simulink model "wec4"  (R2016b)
settings: Solver=ode4  StartTime=0  StopTime=1000  FixedStep=0.005  MaxStep=0.005  RelTol=1e-3  EnableMultiTasking=on
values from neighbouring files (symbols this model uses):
  arAdaptiveLawData = 1/2*zModelSimple.zModelPto.arFreq.*     zModelSimple.zModelPto.arMagnitude./     cos(zModelSimple.zModelPto.arPhase*pi/180+pi/2)    [IMPACT_Control.m]
  arAdaptiveLawDataX = 1/2*zModelSimpleX.zModelPto.arFreq.*         zModelSimpleX.zModelPto.arMagnitude./         cos(zModelSimpleX.zModelPto.arPhase*pi/180+pi/2)    [IMPACT_Control.m]
  arControllerRampGain = [0,0,1,1]    [IMPACT_Control.m]
  arControllerRampTime = [0 rStartRampTime rStartRampTime+rRampTimeLength 8000]    [IMPACT_Control.m]
  arEkfInitialisation = zeros(1,11)    [IMPACT_Control.m]
  arEkfInitialisationX = zeros(1,11)    [IMPACT_Control.m]
  arFrequency = zModelSimple.zModelPto.arFreq    [IMPACT_Control.m]
  arFrequencyRange = zModelSimple.zModelPto.arFreq    [IMPACT_Control.m]
  arFrequencyX = zModelSimpleX.zModelPto.arFreq    [IMPACT_Control.m]
  arImpedance = 1./zModelSimple.zModelPto.arMagnitude./zModelSimple.zModelPto.arFreq    [IMPACT_Control.m]
  arImpedanceX = 1./zModelSimpleX.zModelPto.arMagnitude./zModelSimpleX.zModelPto.arFreq    [IMPACT_Control.m]
  CentralPTOPreload = -1.6113e+07    (= -16113000)    [wecSimInputFile.m]
  F1 = [4.243 2.375 -12.243]    [wecSimInputFile.m]
  F2 = [4.243 -2.375 -12.243]    [wecSimInputFile.m]
  F3 = [-4.243 -2.375 -12.243]    [wecSimInputFile.m]
  F4 = [-4.243 2.375 -12.243]    [wecSimInputFile.m]
  FC = [0 0 -14]    [wecSimInputFile.m]
  iAdaptiveDamping = 0    [wec4IMPACT_Project.m]    (also in IMPACT_Control.m = handles.iAdaptiveDamping; wec1_IMPACT_Project.m; wec2_IMPACT_Project.m; wec3_IMPACT_Project.m)
  iControlType = 2    [wec4IMPACT_Project.m]    (also in IMPACT_Control.m = handles.iControlType; wec1_IMPACT_Project.m = 1; wec2_IMPACT_Project.m = 1; wec3_IMPACT_Project.m = 1)
  iPtoPositionConstraint = 1    [wec4IMPACT_Project.m]    (also in IMPACT_Control.m = handles.iPtoPositionConstraint; wec1_IMPACT_Project.m = 0; wec2_IMPACT_Project.m; wec3_IMPACT_Project.m)
  iSensorNoise = 0    [IMPACT_Control.m]
  m = m+1    (= 2)    [checkParamFile.m]
  PTOrotation = atan((T1(2)-F1(2))/(T1(1)-F1(1)))    [wecSimInputFile.m]
  rCogFloater = -8    [wec4_IMPACT_Model.m]    (also in paramInitial.m = get( handles.edit_rCogFloater, 'String' ); wec1_IMPACT_Model.m = -18; wec2_IMPACT_Model.m = -8.5; wec3_IMPACT_Model.m = -0.7)
  rCogSpar = -36.6    [wec4_IMPACT_Model.m]    (also in paramInitial.m = get( handles.edit_rCogSpar, 'String' ); wec3_IMPACT_Model.m = -21.3; wec3_IMPACT_Model2.m = -21.3)
  rDisplacementLimit = 10.000000    (= 10)    [wec4IMPACT_Project.m]    (also in IMPACT_Control.m = getValue(handles.edit_displacementLimit); wec1_IMPACT_Project.m; wec2_IMPACT_Project.m; wec3_IMPACT_Project.m = 3)
  rDisplacementLimitX = 10.000000    (= 10)    [wec4IMPACT_Project.m]    (also in IMPACT_Control.m = getValue(handles.edit_displacementLimitX); wec1_IMPACT_Project.m = 0; wec2_IMPACT_Project.m; wec3_IMPACT_Project.m = 0)
  rGainForAntiWIndUp = tfControllerDiscrete.rGain    [IMPACT_Control.m]
  rGainForAntiWIndUpX = tfControllerXDiscrete.rGain    [IMPACT_Control.m]
  rMaxForcePto = 300000000.000000    (= 300000000)    [wec4IMPACT_Project.m]    (also in IMPACT_Control.m = getValue(handles.edit_maxForcePto); wec1_IMPACT_Project.m = 1e+15; wec2_IMPACT_Project.m = 1e+15; wec3_IMPACT_Project.m = 1000000000)
  rMinForcePto = -300000000.000000    (= -300000000)    [wec4IMPACT_Project.m]    (also in IMPACT_Control.m = getValue(handles.edit_minForcePto); wec1_IMPACT_Project.m = -1e+15; wec2_IMPACT_Project.m = -1e+15; wec3_IMPACT_Project.m = -1000000000)
  rMooringX = 20000    [wec4_IMPACT_Model.m]    (also in paramInitial.m = get( handles.edit_rMooringX, 'String' ); wec3_IMPACT_Model.m = 10000; wec3_IMPACT_Model2.m = 10000)
  rMooringZ = 10000    [wec4_IMPACT_Model.m]    (also in paramInitial.m = get( handles.edit_rMooringZ, 'String' ); wec3_IMPACT_Model.m = 0; wec3_IMPACT_Model2.m = 0)
  rOutputSampleTime = 0.010000    (= 0.01)    [wec4IMPACT_Project.m]    (also in IMPACT_Control.m = getValue(handles.edit_outputSampleTime); wec1_IMPACT_Project.m; wec2_IMPACT_Project.m; wec3_IMPACT_Project.m)
  rPassiveDampingGain = -604830.000000    (= -604830)    [wec4IMPACT_Project.m]    (also in IMPACT_Control.m = getValue(handles.edit_gainPLD); wec1_IMPACT_Project.m = -214018.1537; wec2_IMPACT_Project.m = -1948070; wec3_IMPACT_Project.m = -519390)
  rPassiveDampingGainX = -278660.000000    (= -278660)    [wec4IMPACT_Project.m]    (also in IMPACT_Control.m = getValue(handles.edit_gainPLDX); wec1_IMPACT_Project.m = 0; wec2_IMPACT_Project.m = 0; wec3_IMPACT_Project.m = 0)
  rTetherPretension = 1.6113e+07    (= 16113000)    [wec4_IMPACT_Model.m]    (also in paramInitial.m = get( handles.edit_rTetherPretension, 'String' ); wec3_IMPACT_Model.m = 0; wec3_IMPACT_Model2.m = 0)
  rTetherSpring = 500000    [wec4_IMPACT_Model.m]    (also in paramInitial.m = get( handles.edit_rTetherSpring, 'String' ); wec3_IMPACT_Model.m = 0; wec3_IMPACT_Model2.m = 0)
  rUpperFrequencyLimit = EKFFloater.upperFreq    [IMPACT_Control.m]
  rXf = 4.243    [wec4AdditionalParams.m]
  rXs = 16.075    [wec4AdditionalParams.m]
  rYf = 2.375    [wec4AdditionalParams.m]
  rYs = 16.075    [wec4AdditionalParams.m]
  rZf = 4.243    [wec4AdditionalParams.m]
  rZs = 2.4350    (= 2.435)    [wec4AdditionalParams.m]
  rZTetherF = 6    [wec4AdditionalParams.m]
  rZTetherS = 2.4350    (= 2.435)    [wec4AdditionalParams.m]
  s = tf('s')    [wec4_IMPACT_Model.m]    (also in IMPACT_Control.m; wec1_IMPACT_Model.m; wec2_IMPACT_Model.m; wec3_IMPACT_Model.m)
  SidePTO1Preload = PreloadPTOCorner    (= 0)    [wecSimInputFile.m]
  SidePTO2Preload = PreloadPTOCorner    (= 0)    [wecSimInputFile.m]
  SidePTO3Preload = PreloadPTOCorner    (= 0)    [wecSimInputFile.m]
  SidePTO4Preload = PreloadPTOCorner    (= 0)    [wecSimInputFile.m]
  simu = simulationClass()    [wecSimInputFile.m]
  T1 = [16.075 16.075 -34.165]    [wecSimInputFile.m]
  T2 = [16.075 -16.075 -34.165]    [wecSimInputFile.m]
  T3 = [-16.075 -16.075 -34.165]    [wecSimInputFile.m]
  T4 = [-16.075 16.075 -34.165]    [wecSimInputFile.m]
  TC = [0 0 -34.165]    [wecSimInputFile.m]
  waves = waveClass('irregular')    [wecSimInputFile.m]
  Z = magPhaseToComplex(zModelTf)    [IMPACT_Control.m]
undefined symbols (not defined in the file or in its folder): arControllerDiscreteDen, arControllerDiscreteNum, arControllerDiscreteXDen, arControllerDiscreteXNum, arExcForceFloaterDen, arExcForceFloaterNum, arExcForceFloaterXDen, arExcForceFloaterXNum, arExcForceSparDen, arExcForceSparNum, arExcForceSparXDen, arExcForceSparXNum, arFexcFloaterDen, arFexcFloaterNum, arFexcFloaterXDen, arFexcFloaterXNum, arFexcSparDen, arFexcSparNum, arFexcSparXDen, arFexcSparXNum, Body, body, constraint, CTTime, deg, Elements, geometry, IRKB, kg, lenJ, mooring, N, pto, rAccelerationGainFloater, rAccelerationGainFloaterX, rAccelerationGainSpar, rAccelerationGainSparX, rad, rBuoyancyGainFloater, rBuoyancyGainFloaterX, rBuoyancyGainSpar, rBuoyancyGainSparX, rDampingGainFloater, rDampingGainFloaterX, rDampingGainSpar, rDampingGainSparX, Rigid, rMaxFocePto, wec4_float, wec4_reactor, WECSim_Lib, X, Y
libraries: nesl_utility x380, sm_lib x170, vrlib x91, simulink x12, WECSim_Lib x4
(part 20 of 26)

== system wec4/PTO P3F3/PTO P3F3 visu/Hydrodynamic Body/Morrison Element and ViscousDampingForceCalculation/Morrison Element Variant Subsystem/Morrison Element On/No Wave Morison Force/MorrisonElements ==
  r : Inport  Partition=on  PartitionDimension=1  PartitionWidth=1
  Vel : Inport  Port=2
  Accel : Inport  Port=3
  Disp : Inport  Port=4
  Area : Inport  Port=5  Partition=on  PartitionDimension=1  PartitionWidth=1
  Cd : Inport  Port=6  Partition=on  PartitionDimension=1  PartitionWidth=1
  Vol : Inport  Port=7  Partition=on  PartitionDimension=1  PartitionWidth=1
  Ca : Inport  Port=8  Partition=on  PartitionDimension=1  PartitionWidth=1
  Time : Inport  Port=9
  3x3 : Concatenate  NumInputs=3  Mode=Multidimensional array
  A x 3x3 : Product  Multiplication=Matrix(*)
  Accel-sl : Selector  InputPortWidth=6  IndexOptions=Index vector (dialog)  Indices=[1 2 3]  OutputSizes=1
  Accel-sr : Selector  InputPortWidth=6  IndexOptions=Index vector (dialog)  Indices=[4 5 6]  OutputSizes=1
  AccelDiff-u : Sum  Inputs=+-
  AccelDiff-v : Sum  Inputs=+-
  AccelDiff-w : Sum  Inputs=+-
  Add Accel : Sum  Inputs=+++
  Add Vel : Sum
  Ax : Selector  InputPortWidth=3  IndexOptions=Index vector (dialog)  Indices=[1]  OutputSizes=1
  Ay : Selector  InputPortWidth=3  IndexOptions=Index vector (dialog)  Indices=[2]  OutputSizes=1
  Az : Selector  InputPortWidth=3  IndexOptions=Index vector (dialog)  Indices=[3]  OutputSizes=1
  Cax : Selector  InputPortWidth=3  IndexOptions=Index vector (dialog)  Indices=[1]  OutputSizes=1
  Cay : Selector  InputPortWidth=3  IndexOptions=Index vector (dialog)  Indices=[2]  OutputSizes=1
  Caz : Selector  InputPortWidth=3  IndexOptions=Index vector (dialog)  Indices=[3]  OutputSizes=1
  Cdx : Selector  InputPortWidth=3  IndexOptions=Index vector (dialog)  Indices=[1]  OutputSizes=1
  Cdy : Selector  InputPortWidth=3  IndexOptions=Index vector (dialog)  Indices=[2]  OutputSizes=1
  Cdz : Selector  InputPortWidth=3  IndexOptions=Index vector (dialog)  Indices=[3]  OutputSizes=1
  Constant : Constant  Value=0
  Density : Constant  Value=simu.rho
  Disp-sl : Selector  InputPortWidth=6  IndexOptions=Index vector (dialog)  Indices=[1 2 3]  OutputSizes=1
  Disp-sr : Selector  InputPortWidth=6  IndexOptions=Index vector (dialog)  Indices=[4 5 6]  OutputSizes=1
  For Each : ForEach  DisableCoverage=on  IndexMode=One-based
  ForceCom : Concatenate  NumInputs=3  ConcatenateDimension=2
  Fout : Concatenate  NumInputs=6  Mode=Multidimensional array  ConcatenateDimension=2
  Fx-A : Product  Inputs=4
  Fx-AFK : Product  Inputs=3
  Fx-Sum : Sum  Inputs=+++
  Fx-V : Product  Inputs=5
  Fx-V1 : Product  Inputs=5
  Fy-A : Product  Inputs=4
  Fy-AFK : Product  Inputs=3
  Fy-Sum : Sum  Inputs=+++
  Fz-A : Product  Inputs=4
  Fz-AFK : Product  Inputs=3
  Fz-Sum : Sum  Inputs=+++
  Fz-w : Product  Inputs=5
  Mx : Selector  InputPortWidth=3  IndexOptions=Index vector (dialog)  Indices=[1]  OutputSizes=1
  My : Selector  InputPortWidth=3  IndexOptions=Index vector (dialog)  Indices=[2]  OutputSizes=1
  Mz : Selector  InputPortWidth=3  IndexOptions=Index vector (dialog)  Indices=[3]  OutputSizes=1
  OrbitalVelocity : Subsystem
  Rotation1 : Subsystem
  Rotation2 : Subsystem
  Rotation3 : Subsystem
  ShiftCg : Sum
  SwitchFx : Switch  Criteria=u2 > Threshold
  SwitchFy : Switch  Criteria=u2 > Threshold
  SwitchFz : Switch  Criteria=u2 > Threshold
  Ux : Selector  InputPortWidth=3  IndexOptions=Index vector (dialog)  Indices=[1]  OutputSizes=1
  Uy : Selector  InputPortWidth=3  IndexOptions=Index vector (dialog)  Indices=[2]  OutputSizes=1
  Uz : Selector  InputPortWidth=3  IndexOptions=Index vector (dialog)  Indices=[3]  OutputSizes=1
  V-u : Abs
  V-v : Abs
  V-w : Abs
  V^2-u : Product
  V^2-v : Product
  V^2-w : Product
  Vel-sl : Selector  InputPortWidth=6  IndexOptions=Index vector (dialog)  Indices=[1 2 3]  OutputSizes=1
  "Vel-sr " : Selector  InputPortWidth=6  IndexOptions=Index vector (dialog)  Indices=[4 5 6]  OutputSizes=1
  VelDiff-u : Sum  Inputs=+-
  VelDiff-v : Sum  Inputs=+-
  VelDiff-w : Sum  Inputs=+-
  Zshift : Selector  InputPortWidth=3  IndexOptions=Index vector (dialog)  Indices=[3]  OutputSizes=1
  abs-Area : Abs
  abs-Ca : Abs
  abs-Cd : Abs
  "dot{U}x" : Selector  InputPortWidth=3  IndexOptions=Index vector (dialog)  Indices=[1]  OutputSizes=1
  "dot{U}y" : Selector  InputPortWidth=3  IndexOptions=Index vector (dialog)  Indices=[2]  OutputSizes=1
  "dot{U}z" : Selector  InputPortWidth=3  IndexOptions=Index vector (dialog)  Indices=[3]  OutputSizes=1
  "dot{w} x r2" : vrlib/Utilities/Cross Product
  half : Constant  Value=1/2
  r x 3x1 : Product  Multiplication=Matrix(*)
  r x 3x2 : Product  Multiplication=Matrix(*)
  r x 3x3 : Product  Multiplication=Matrix(*)
  "r_{cg} x F" : vrlib/Utilities/Cross Product
  rot1 : Selector  InputPortWidth=3  IndexOptions=Index vector (dialog)  Indices=[1]  OutputSizes=1
  rot2 : Selector  InputPortWidth=3  IndexOptions=Index vector (dialog)  Indices=[2]  OutputSizes=1
  rot3 : Selector  InputPortWidth=3  IndexOptions=Index vector (dialog)  Indices=[3]  OutputSizes=1
  w x r : vrlib/Utilities/Cross Product
  w x w x r : vrlib/Utilities/Cross Product
  Force : Outport  PortDimensions=[1 6]  ConcatenationDimension=1
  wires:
  Time/1 -> OrbitalVelocity/2(Time)
  abs-Cd/1 -> r x 3x1/1
  abs-Ca/1 -> Caz/1, Cay/1, Cax/1
  V-w/1 -> V^2-w/1
  Constant/1 -> SwitchFx/1, SwitchFz/1, SwitchFy/1
  Fx-V1/1 -> Fy-Sum/1
  Fy-A/1 -> Fy-Sum/2
  Cay/1 -> Fy-A/4
  AccelDiff-v/1 -> Fy-A/1
  Fy-AFK/1 -> Fy-Sum/3
  Fy-Sum/1 -> SwitchFy/3
  SwitchFy/1 -> ForceCom/2, Fout/2
  Cdy/1 -> Fx-V1/4
  Ay/1 -> Fx-V1/5
  OrbitalVelocity/5(v-V) -> VelDiff-v/1
  VelDiff-v/1 -> V^2-v/2, V-v/1
  V-v/1 -> V^2-v/1
  V^2-v/1 -> Fx-V1/1
  OrbitalVelocity/6(v-A) -> Fy-AFK/1, AccelDiff-v/1
  r x 3x2/1 -> abs-Ca/1
  Ca/1 -> r x 3x2/1
  r x 3x1/1 -> Cdx/1, Cdz/1, Cdy/1
  Cd/1 -> abs-Cd/1
  Cax/1 -> Fx-A/4
  Caz/1 -> Fz-A/4
  Fout/1 -> Force/1
  ForceCom/1 -> "r_{cg} x F"/2
  abs-Area/1 -> Ax/1, Az/1, Ay/1
  A x 3x3/1 -> abs-Area/1
  Cdz/1 -> Fz-w/4
  Cdx/1 -> Fx-V/4
  Ax/1 -> Fx-V/5
  Area/1 -> A x 3x3/1
  Az/1 -> Fz-w/5
  Fz-Sum/1 -> SwitchFz/3
  Fx-Sum/1 -> SwitchFx/3
  SwitchFx/1 -> ForceCom/1, Fout/1
  SwitchFz/1 -> Fout/3, ForceCom/3
  Zshift/1 -> SwitchFz/2, SwitchFx/2, SwitchFy/2
  VelDiff-u/1 -> V^2-u/2, V-u/1
  V-u/1 -> V^2-u/1
  3x3/1 -> r x 3x1/2, r x 3x2/2, r x 3x3/2, A x 3x3/2
  Mz/1 -> Fout/6
  My/1 -> Fout/5
  Mx/1 -> Fout/4
  "r_{cg} x F"/1 -> Mx/1, My/1, Mz/1
  Fz-AFK/1 -> Fz-Sum/3
  Fz-A/1 -> Fz-Sum/2
  Fz-w/1 -> Fz-Sum/1
  Fx-AFK/1 -> Fx-Sum/3
  Fx-A/1 -> Fx-Sum/2
  Fx-V/1 -> Fx-Sum/1
  OrbitalVelocity/4(w-A) -> AccelDiff-w/1, Fz-AFK/1
  AccelDiff-w/1 -> Fz-A/1
  Vol/1 -> Fx-A/3, Fz-A/2, Fx-AFK/2, Fz-AFK/2, Fy-AFK/2, Fy-A/2
  AccelDiff-u/1 -> Fx-A/1
  V^2-w/1 -> Fz-w/1
  Density/1 -> Fx-V/3, Fx-V1/3, Fz-w/3, Fx-A/2, Fz-A/3, Fx-AFK/3, Fz-AFK/3, Fy-AFK/3, Fy-A/3
  half/1 -> Fx-V/2, Fx-V1/2, Fz-w/2
  V^2-u/1 -> Fx-V/1
  VelDiff-w/1 -> V^2-w/2, V-w/1
  OrbitalVelocity/2(w-V) -> VelDiff-w/1
  OrbitalVelocity/1(u-V) -> VelDiff-u/1
  Uz/1 -> VelDiff-w/2
  Ux/1 -> VelDiff-u/2
  Uy/1 -> VelDiff-v/2
  Add Vel/1 -> Ux/1, Uz/1, Uy/1
  "dot{U}z"/1 -> AccelDiff-w/2
  OrbitalVelocity/3(u-A) -> Fx-AFK/1, AccelDiff-u/1
  "dot{U}x"/1 -> AccelDiff-u/2
  "dot{U}y"/1 -> AccelDiff-v/2
  ShiftCg/1 -> OrbitalVelocity/1(Disp), Zshift/1
  Disp-sl/1 -> ShiftCg/2
  r x 3x3/1 -> ShiftCg/1, "r_{cg} x F"/1
  Rotation3/1(rot[3,1-3]) -> 3x3/3
  Rotation1/1(rot[1,1-3]) -> 3x3/1
  Rotation2/1(rot[2,1-3]) -> 3x3/2
  rot2/1 -> Rotation1/2(rot2), Rotation2/2(rot2), Rotation3/2(rot2)
  rot1/1 -> Rotation1/1(rot1), Rotation2/1(rot1), Rotation3/1(rot1)
  rot3/1 -> Rotation1/3(rot3), Rotation2/3(rot3)
  Disp-sr/1 -> rot1/1, rot2/1, rot3/1
  Disp/1 -> Disp-sr/1, Disp-sl/1
  Vel-sl/1 -> Add Vel/1
  Add Accel/1 -> "dot{U}x"/1, "dot{U}y"/1, "dot{U}z"/1
  Accel-sl/1 -> Add Accel/3
  "dot{w} x r2"/1 -> Add Accel/2
  Accel-sr/1 -> "dot{w} x r2"/1
  Accel/1 -> Accel-sr/1, Accel-sl/1
  r/1 -> w x r/2, "dot{w} x r2"/2, r x 3x3/1
  "Vel-sr "/1 -> w x r/1, w x w x r/1
  w x w x r/1 -> Add Accel/1
  w x r/1 -> w x w x r/2, Add Vel/2
  Vel/1 -> "Vel-sr "/1, Vel-sl/1

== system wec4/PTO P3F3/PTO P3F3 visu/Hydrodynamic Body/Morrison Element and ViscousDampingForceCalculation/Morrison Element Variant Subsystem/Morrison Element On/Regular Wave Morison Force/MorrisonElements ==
  r : Inport  Partition=on  PartitionDimension=1  PartitionWidth=1
  Vel : Inport  Port=2
  Accel : Inport  Port=3
  Disp : Inport  Port=4
  Area : Inport  Port=5  Partition=on  PartitionDimension=1  PartitionWidth=1
  Cd : Inport  Port=6  Partition=on  PartitionDimension=1  PartitionWidth=1
  Vol : Inport  Port=7  Partition=on  PartitionDimension=1  PartitionWidth=1
  Ca : Inport  Port=8  Partition=on  PartitionDimension=1  PartitionWidth=1
  Time : Inport  Port=9
  3x3 : Concatenate  NumInputs=3  Mode=Multidimensional array
  A x 3x3 : Product  Multiplication=Matrix(*)
  Accel-sl : Selector  InputPortWidth=6  IndexOptions=Index vector (dialog)  Indices=[1 2 3]  OutputSizes=1
  Accel-sr : Selector  InputPortWidth=6  IndexOptions=Index vector (dialog)  Indices=[4 5 6]  OutputSizes=1
  AccelDiff-u : Sum  Inputs=+-
  AccelDiff-v : Sum  Inputs=+-
  AccelDiff-w : Sum  Inputs=+-
  Add Accel : Sum  Inputs=+++
  Add Vel : Sum
  Ax : Selector  InputPortWidth=3  IndexOptions=Index vector (dialog)  Indices=[1]  OutputSizes=1
  Ay : Selector  InputPortWidth=3  IndexOptions=Index vector (dialog)  Indices=[2]  OutputSizes=1
  Az : Selector  InputPortWidth=3  IndexOptions=Index vector (dialog)  Indices=[3]  OutputSizes=1
  Cax : Selector  InputPortWidth=3  IndexOptions=Index vector (dialog)  Indices=[1]  OutputSizes=1
  Cay : Selector  InputPortWidth=3  IndexOptions=Index vector (dialog)  Indices=[2]  OutputSizes=1
  Caz : Selector  InputPortWidth=3  IndexOptions=Index vector (dialog)  Indices=[3]  OutputSizes=1
  Cdx : Selector  InputPortWidth=3  IndexOptions=Index vector (dialog)  Indices=[1]  OutputSizes=1
  Cdy : Selector  InputPortWidth=3  IndexOptions=Index vector (dialog)  Indices=[2]  OutputSizes=1
  Cdz : Selector  InputPortWidth=3  IndexOptions=Index vector (dialog)  Indices=[3]  OutputSizes=1
  Constant : Constant  Value=0
  Density : Constant  Value=simu.rho
  Disp-sl : Selector  InputPortWidth=6  IndexOptions=Index vector (dialog)  Indices=[1 2 3]  OutputSizes=1
  Disp-sr : Selector  InputPortWidth=6  IndexOptions=Index vector (dialog)  Indices=[4 5 6]  OutputSizes=1
  For Each : ForEach  DisableCoverage=on  IndexMode=One-based
  ForceCom : Concatenate  NumInputs=3  ConcatenateDimension=2
  Fout : Concatenate  NumInputs=6  Mode=Multidimensional array  ConcatenateDimension=2
  Fx-A : Product  Inputs=4
  Fx-AFK : Product  Inputs=3
  Fx-Sum : Sum  Inputs=+++
  Fx-V : Product  Inputs=5
  Fx-V1 : Product  Inputs=5
  Fy-A : Product  Inputs=4
  Fy-AFK : Product  Inputs=3
  Fy-Sum : Sum  Inputs=+++
  Fz-A : Product  Inputs=4
  Fz-AFK : Product  Inputs=3
  Fz-Sum : Sum  Inputs=+++
  Fz-w : Product  Inputs=5
  Mx : Selector  InputPortWidth=3  IndexOptions=Index vector (dialog)  Indices=[1]  OutputSizes=1
  My : Selector  InputPortWidth=3  IndexOptions=Index vector (dialog)  Indices=[2]  OutputSizes=1
  Mz : Selector  InputPortWidth=3  IndexOptions=Index vector (dialog)  Indices=[3]  OutputSizes=1
  OrbitalVelocity : Subsystem
  Rotation1 : Subsystem
  Rotation2 : Subsystem
  Rotation3 : Subsystem
  ShiftCg : Sum
  SwitchFx : Switch  Criteria=u2 > Threshold
  SwitchFy : Switch  Criteria=u2 > Threshold
  SwitchFz : Switch  Criteria=u2 > Threshold
  Ux : Selector  InputPortWidth=3  IndexOptions=Index vector (dialog)  Indices=[1]  OutputSizes=1
  Uy : Selector  InputPortWidth=3  IndexOptions=Index vector (dialog)  Indices=[2]  OutputSizes=1
  Uz : Selector  InputPortWidth=3  IndexOptions=Index vector (dialog)  Indices=[3]  OutputSizes=1
  V-u : Abs
  V-v : Abs
  V-w : Abs
  V^2-u : Product
  V^2-v : Product
  V^2-w : Product
  Vel-sl : Selector  InputPortWidth=6  IndexOptions=Index vector (dialog)  Indices=[1 2 3]  OutputSizes=1
  "Vel-sr " : Selector  InputPortWidth=6  IndexOptions=Index vector (dialog)  Indices=[4 5 6]  OutputSizes=1
  VelDiff-u : Sum  Inputs=+-
  VelDiff-v : Sum  Inputs=+-
  VelDiff-w : Sum  Inputs=+-
  Zshift : Selector  InputPortWidth=3  IndexOptions=Index vector (dialog)  Indices=[3]  OutputSizes=1
  abs-Area : Abs
  abs-Ca : Abs
  abs-Cd : Abs
  "dot{U}x" : Selector  InputPortWidth=3  IndexOptions=Index vector (dialog)  Indices=[1]  OutputSizes=1
  "dot{U}y" : Selector  InputPortWidth=3  IndexOptions=Index vector (dialog)  Indices=[2]  OutputSizes=1
  "dot{U}z" : Selector  InputPortWidth=3  IndexOptions=Index vector (dialog)  Indices=[3]  OutputSizes=1
  "dot{w} x r2" : vrlib/Utilities/Cross Product
  half : Constant  Value=1/2
  r x 3x1 : Product  Multiplication=Matrix(*)
  r x 3x2 : Product  Multiplication=Matrix(*)
  r x 3x3 : Product  Multiplication=Matrix(*)
  "r_{cg} x F" : vrlib/Utilities/Cross Product
  rot1 : Selector  InputPortWidth=3  IndexOptions=Index vector (dialog)  Indices=[1]  OutputSizes=1
  rot2 : Selector  InputPortWidth=3  IndexOptions=Index vector (dialog)  Indices=[2]  OutputSizes=1
  rot3 : Selector  InputPortWidth=3  IndexOptions=Index vector (dialog)  Indices=[3]  OutputSizes=1
  w x r : vrlib/Utilities/Cross Product
  w x w x r : vrlib/Utilities/Cross Product
  Force : Outport  PortDimensions=[1 6]  ConcatenationDimension=1
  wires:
  Time/1 -> OrbitalVelocity/2(Time)
  abs-Cd/1 -> r x 3x1/1
  abs-Ca/1 -> Caz/1, Cay/1, Cax/1
  V-w/1 -> V^2-w/1
  Constant/1 -> SwitchFx/1, SwitchFz/1, SwitchFy/1
  Fx-V1/1 -> Fy-Sum/1
  Fy-A/1 -> Fy-Sum/2
  Cay/1 -> Fy-A/4
  AccelDiff-v/1 -> Fy-A/1
  Fy-AFK/1 -> Fy-Sum/3
  Fy-Sum/1 -> SwitchFy/3
  SwitchFy/1 -> ForceCom/2, Fout/2
  Cdy/1 -> Fx-V1/4
  Ay/1 -> Fx-V1/5
  OrbitalVelocity/5(v-V) -> VelDiff-v/1
  VelDiff-v/1 -> V^2-v/2, V-v/1
  V-v/1 -> V^2-v/1
  V^2-v/1 -> Fx-V1/1
  OrbitalVelocity/6(v-A) -> Fy-AFK/1, AccelDiff-v/1
  r x 3x2/1 -> abs-Ca/1
  Ca/1 -> r x 3x2/1
  r x 3x1/1 -> Cdx/1, Cdz/1, Cdy/1
  Cd/1 -> abs-Cd/1
  Cax/1 -> Fx-A/4
  Caz/1 -> Fz-A/4
  Fout/1 -> Force/1
  ForceCom/1 -> "r_{cg} x F"/2
  abs-Area/1 -> Ax/1, Az/1, Ay/1
  A x 3x3/1 -> abs-Area/1
  Cdz/1 -> Fz-w/4
  Cdx/1 -> Fx-V/4
  Ax/1 -> Fx-V/5
  Area/1 -> A x 3x3/1
  Az/1 -> Fz-w/5
  Fz-Sum/1 -> SwitchFz/3
  Fx-Sum/1 -> SwitchFx/3
  SwitchFx/1 -> ForceCom/1, Fout/1
  SwitchFz/1 -> Fout/3, ForceCom/3
  Zshift/1 -> SwitchFz/2, SwitchFx/2, SwitchFy/2
  VelDiff-u/1 -> V^2-u/2, V-u/1
  V-u/1 -> V^2-u/1
  3x3/1 -> r x 3x1/2, r x 3x2/2, r x 3x3/2, A x 3x3/2
  Mz/1 -> Fout/6
  My/1 -> Fout/5
  Mx/1 -> Fout/4
  "r_{cg} x F"/1 -> Mx/1, My/1, Mz/1
  Fz-AFK/1 -> Fz-Sum/3
  Fz-A/1 -> Fz-Sum/2
  Fz-w/1 -> Fz-Sum/1
  Fx-AFK/1 -> Fx-Sum/3
  Fx-A/1 -> Fx-Sum/2
  Fx-V/1 -> Fx-Sum/1
  OrbitalVelocity/4(w-A) -> AccelDiff-w/1, Fz-AFK/1
  AccelDiff-w/1 -> Fz-A/1
  Vol/1 -> Fx-A/3, Fz-A/2, Fx-AFK/2, Fz-AFK/2, Fy-AFK/2, Fy-A/2
  AccelDiff-u/1 -> Fx-A/1
  V^2-w/1 -> Fz-w/1
  Density/1 -> Fx-V/3, Fx-V1/3, Fz-w/3, Fx-A/2, Fz-A/3, Fx-AFK/3, Fz-AFK/3, Fy-AFK/3, Fy-A/3
  half/1 -> Fx-V/2, Fx-V1/2, Fz-w/2
  V^2-u/1 -> Fx-V/1
  VelDiff-w/1 -> V^2-w/2, V-w/1
  OrbitalVelocity/2(w-V) -> VelDiff-w/1
  OrbitalVelocity/1(u-V) -> VelDiff-u/1
  Uz/1 -> VelDiff-w/2
  Ux/1 -> VelDiff-u/2
  Uy/1 -> VelDiff-v/2
  Add Vel/1 -> Ux/1, Uz/1, Uy/1
  "dot{U}z"/1 -> AccelDiff-w/2
  OrbitalVelocity/3(u-A) -> Fx-AFK/1, AccelDiff-u/1
  "dot{U}x"/1 -> AccelDiff-u/2
  "dot{U}y"/1 -> AccelDiff-v/2
  ShiftCg/1 -> OrbitalVelocity/1(Disp), Zshift/1
  Disp-sl/1 -> ShiftCg/2
  r x 3x3/1 -> ShiftCg/1, "r_{cg} x F"/1
  Rotation3/1(rot[3,1-3]) -> 3x3/3
  Rotation1/1(rot[1,1-3]) -> 3x3/1
  Rotation2/1(rot[2,1-3]) -> 3x3/2
  rot2/1 -> Rotation1/2(rot2), Rotation2/2(rot2), Rotation3/2(rot2)
  rot1/1 -> Rotation1/1(rot1), Rotation2/1(rot1), Rotation3/1(rot1)
  rot3/1 -> Rotation1/3(rot3), Rotation2/3(rot3)
  Disp-sr/1 -> rot1/1, rot2/1, rot3/1
  Disp/1 -> Disp-sr/1, Disp-sl/1
  Vel-sl/1 -> Add Vel/1
  Add Accel/1 -> "dot{U}x"/1, "dot{U}y"/1, "dot{U}z"/1
  Accel-sl/1 -> Add Accel/3
  "dot{w} x r2"/1 -> Add Accel/2
  Accel-sr/1 -> "dot{w} x r2"/1
  Accel/1 -> Accel-sr/1, Accel-sl/1
  r/1 -> w x r/2, "dot{w} x r2"/2, r x 3x3/1
  "Vel-sr "/1 -> w x r/1, w x w x r/1
  w x w x r/1 -> Add Accel/1
  w x r/1 -> w x w x r/2, Add Vel/2
  Vel/1 -> "Vel-sr "/1, Vel-sl/1

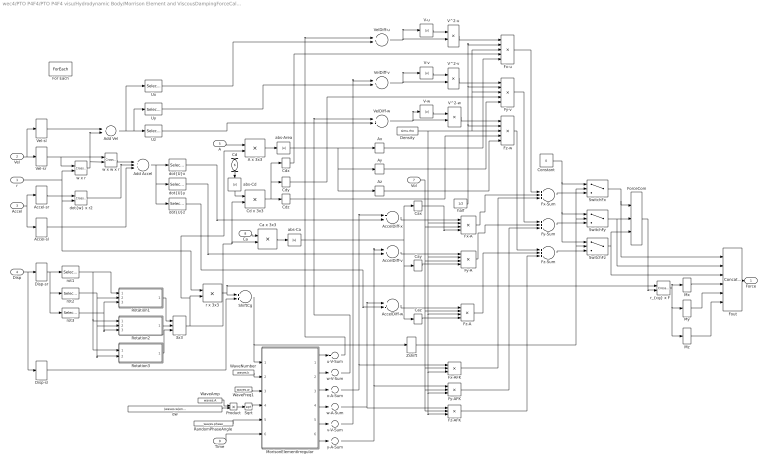
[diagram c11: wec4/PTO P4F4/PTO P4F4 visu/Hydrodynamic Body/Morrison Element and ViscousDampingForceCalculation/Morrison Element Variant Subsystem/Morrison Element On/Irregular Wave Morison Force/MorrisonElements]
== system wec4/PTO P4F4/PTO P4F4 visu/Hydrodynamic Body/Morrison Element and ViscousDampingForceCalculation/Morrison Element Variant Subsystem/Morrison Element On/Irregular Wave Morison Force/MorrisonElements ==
  r : Inport  Partition=on  PartitionDimension=1  PartitionWidth=1
  Vel : Inport  Port=2
  Accel : Inport  Port=3
  Disp : Inport  Port=4
  A : Inport  Port=5  Partition=on  PartitionDimension=1  PartitionWidth=1
  Cd : Inport  Port=6  Partition=on  PartitionDimension=1  PartitionWidth=1
  Vol : Inport  Port=7  Partition=on  PartitionDimension=1  PartitionWidth=1
  Ca : Inport  Port=8  Partition=on  PartitionDimension=1  PartitionWidth=1
  Time : Inport  Port=9
  3x3 : Concatenate  NumInputs=3  Mode=Multidimensional array
  A x 3x3 : Product  Multiplication=Matrix(*)
  Accel-sl : Selector  InputPortWidth=6  IndexOptions=Index vector (dialog)  Indices=[1 2 3]  OutputSizes=1
  Accel-sr : Selector  InputPortWidth=6  IndexOptions=Index vector (dialog)  Indices=[4 5 6]  OutputSizes=1
  AccelDiff-v : Sum  Inputs=+-
  AccelDiff-w : Sum  Inputs=+-
  AccelDiff-x : Sum  Inputs=+-
  Add Accel : Sum  Inputs=+++
  Add Vel : Sum
  Ax : Selector  InputPortWidth=3  IndexOptions=Index vector (dialog)  Indices=[1]  OutputSizes=1
  Ay : Selector  InputPortWidth=3  IndexOptions=Index vector (dialog)  Indices=[2]  OutputSizes=1
  Az : Selector  InputPortWidth=3  IndexOptions=Index vector (dialog)  Indices=[3]  OutputSizes=1
  Ca x 3x3 : Product  Multiplication=Matrix(*)
  Cax : Selector  InputPortWidth=3  IndexOptions=Index vector (dialog)  Indices=[1]  OutputSizes=1
  Cay : Selector  InputPortWidth=3  IndexOptions=Index vector (dialog)  Indices=[2]  OutputSizes=1
  Caz : Selector  InputPortWidth=3  IndexOptions=Index vector (dialog)  Indices=[3]  OutputSizes=1
  Cd x 3x3 : Product  Multiplication=Matrix(*)
  Cdx : Selector  InputPortWidth=3  IndexOptions=Index vector (dialog)  Indices=[1]  OutputSizes=1
  Cdy : Selector  InputPortWidth=3  IndexOptions=Index vector (dialog)  Indices=[2]  OutputSizes=1
  Cdz : Selector  InputPortWidth=3  IndexOptions=Index vector (dialog)  Indices=[3]  OutputSizes=1
  Constant : Constant  Value=0
  Density : Constant  Value=simu.rho
  Disp-sl : Selector  InputPortWidth=6  IndexOptions=Index vector (dialog)  Indices=[1 2 3]  OutputSizes=1
  Disp-sr : Selector  InputPortWidth=6  IndexOptions=Index vector (dialog)  Indices=[4 5 6]  OutputSizes=1
  For Each : ForEach  DisableCoverage=on  IndexMode=One-based
  ForceCom : Concatenate  NumInputs=3  ConcatenateDimension=2
  Fout : Concatenate  NumInputs=6  Mode=Multidimensional array  ConcatenateDimension=2
  Fx-A : Product  Inputs=4
  Fx-AFK : Product  Inputs=3
  Fx-Sum : Sum  Inputs=+++
  Fx-u : Product  Inputs=5
  Fy-A : Product  Inputs=4
  Fy-AFK : Product  Inputs=3
  Fy-Sum : Sum  Inputs=+++
  Fy-v : Product  Inputs=5
  Fz-A : Product  Inputs=4
  Fz-AFK : Product  Inputs=3
  Fz-Sum : Sum  Inputs=+++
  Fz-w : Product  Inputs=5
  MorisonElementIrregular : Subsystem  TreatAsAtomicUnit=on
  Mx : Selector  InputPortWidth=3  IndexOptions=Index vector (dialog)  Indices=[1]  OutputSizes=1
  My : Selector  InputPortWidth=3  IndexOptions=Index vector (dialog)  Indices=[2]  OutputSizes=1
  Mz : Selector  InputPortWidth=3  IndexOptions=Index vector (dialog)  Indices=[3]  OutputSizes=1
  Product : Product
  RandomPhaseAngle : Constant  Value=waves.phase  VectorParams1D=off
  Rotation1 : Subsystem
  Rotation2 : Subsystem
  Rotation3 : Subsystem
  ShiftCg : Sum
  Sqrt : Sqrt
  SwitchFx : Switch  Criteria=u2 > Threshold
  SwitchFy : Switch  Criteria=u2 > Threshold
  SwitchFz : Switch  Criteria=u2 > Threshold
  Ux : Selector  InputPortWidth=3  IndexOptions=Index vector (dialog)  Indices=[1]  OutputSizes=1
  Uy : Selector  InputPortWidth=3  IndexOptions=Index vector (dialog)  Indices=[2]  OutputSizes=1
  Uz : Selector  InputPortWidth=3  IndexOptions=Index vector (dialog)  Indices=[3]  OutputSizes=1
  V-u : Abs
  V-v : Abs
  V-w : Abs
  V^2-u : Product
  V^2-v : Product
  V^2-w : Product
  Vel-sl : Selector  InputPortWidth=6  IndexOptions=Index vector (dialog)  Indices=[1 2 3]  OutputSizes=1
  "Vel-sr " : Selector  InputPortWidth=6  IndexOptions=Index vector (dialog)  Indices=[4 5 6]  OutputSizes=1
  VelDiff-u : Sum  Inputs=+-
  VelDiff-v : Sum  Inputs=+-
  VelDiff-w : Sum  Inputs=+-
  WaveAmp : Constant  Value=waves.A  VectorParams1D=off
  WaveFreq1 : Constant  Value=waves.w  VectorParams1D=off
  WaveNumber : Constant  Value=waves.k  VectorParams1D=off
  Zshift : Selector  InputPortWidth=3  IndexOptions=Index vector (dialog)  Indices=[3]  OutputSizes=1
  abs-Area : Abs
  abs-Ca : Abs
  abs-Cd : Abs
  "dot{U}x" : Selector  InputPortWidth=3  IndexOptions=Index vector (dialog)  Indices=[1]  OutputSizes=1
  "dot{U}y" : Selector  InputPortWidth=3  IndexOptions=Index vector (dialog)  Indices=[2]  OutputSizes=1
  "dot{U}z" : Selector  InputPortWidth=3  IndexOptions=Index vector (dialog)  Indices=[3]  OutputSizes=1
  "dot{w} x r2" : vrlib/Utilities/Cross Product
  dw : Constant  Value=(waves.w(end)-waves.w(1))/(waves.numFreq-1)  VectorParams1D=off
  half : Constant  Value=1/2
  r x 3x3 : Product  Multiplication=Matrix(*)
  "r_{cg} x F" : vrlib/Utilities/Cross Product
  rot1 : Selector  InputPortWidth=3  IndexOptions=Index vector (dialog)  Indices=[1]  OutputSizes=1
  rot2 : Selector  InputPortWidth=3  IndexOptions=Index vector (dialog)  Indices=[2]  OutputSizes=1
  rot3 : Selector  InputPortWidth=3  IndexOptions=Index vector (dialog)  Indices=[3]  OutputSizes=1
  u-V-Sum : Sum  Inputs=+  CollapseMode=Specified dimension
  v-V-Sum : Sum  Inputs=+  CollapseMode=Specified dimension
  w x r : vrlib/Utilities/Cross Product
  w x w x r : vrlib/Utilities/Cross Product
  w-A-Sum : Sum  Inputs=+  CollapseMode=Specified dimension
  w-V-Sum : Sum  Inputs=+  CollapseMode=Specified dimension
  x-A-Sum : Sum  Inputs=+  CollapseMode=Specified dimension
  y-A-Sum : Sum  Inputs=+  CollapseMode=Specified dimension
  Force : Outport  PortDimensions=[1 6]  ConcatenationDimension=1
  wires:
  Time/1 -> MorisonElementIrregular/6(Time)
  abs-Cd/1 -> Cd x 3x3/1
  abs-Ca/1 -> Cay/1, Caz/1, Cax/1
  Fy-AFK/1 -> Fy-Sum/3
  Fy-A/1 -> Fy-Sum/2
  AccelDiff-v/1 -> Fy-A/1
  Cay/1 -> Fy-A/4
  y-A-Sum/1 -> AccelDiff-v/1, Fy-AFK/1
  Fy-v/1 -> Fy-Sum/1
  Fy-Sum/1 -> SwitchFy/3
  SwitchFy/1 -> ForceCom/2, Fout/2
  Cdy/1 -> Fy-v/4
  Ay/1 -> Fy-v/5
  V^2-v/1 -> Fy-v/1
  v-V-Sum/1 -> VelDiff-v/1
  V-v/1 -> V^2-v/1
  VelDiff-v/1 -> V^2-v/2, V-v/1
  V-w/1 -> V^2-w/1
  MorisonElementIrregular/6(y-A) -> y-A-Sum/1
  MorisonElementIrregular/5(v-V) -> v-V-Sum/1
  V-u/1 -> V^2-u/1
  MorisonElementIrregular/4(w-A) -> w-A-Sum/1
  MorisonElementIrregular/3(x-A) -> x-A-Sum/1
  MorisonElementIrregular/2(w-V) -> w-V-Sum/1
  Sqrt/1 -> MorisonElementIrregular/4(waves.A)
  Product/1 -> Sqrt/1
  dw/1 -> Product/2
  WaveAmp/1 -> Product/1
  MorisonElementIrregular/1(u-V) -> u-V-Sum/1
  RandomPhaseAngle/1 -> MorisonElementIrregular/5(waves.Phase)
  WaveFreq1/1 -> MorisonElementIrregular/3(waves.w)
  WaveNumber/1 -> MorisonElementIrregular/2(waves.kirr)
  Ca x 3x3/1 -> abs-Ca/1
  Ca/1 -> Ca x 3x3/1
  Cd x 3x3/1 -> Cdx/1, Cdy/1, Cdz/1
  Cd/1 -> abs-Cd/1
  Cax/1 -> Fx-A/4
  Caz/1 -> Fz-A/4
  Fout/1 -> Force/1
  ForceCom/1 -> "r_{cg} x F"/2
  abs-Area/1 -> Ax/1, Az/1, Ay/1
  A x 3x3/1 -> abs-Area/1
  Cdz/1 -> Fz-w/4
  Cdx/1 -> Fx-u/4
  Ax/1 -> Fx-u/5
  A/1 -> A x 3x3/1
  Az/1 -> Fz-w/5
  Fz-Sum/1 -> SwitchFz/3
  Fx-Sum/1 -> SwitchFx/3
  SwitchFx/1 -> ForceCom/1, Fout/1
  SwitchFz/1 -> Fout/3, ForceCom/3
  Zshift/1 -> SwitchFz/2, SwitchFx/2, SwitchFy/2
  VelDiff-u/1 -> V^2-u/2, V-u/1
  3x3/1 -> Cd x 3x3/2, Ca x 3x3/2, r x 3x3/2, A x 3x3/2
  Mz/1 -> Fout/6
  My/1 -> Fout/5
  Mx/1 -> Fout/4
  "r_{cg} x F"/1 -> Mx/1, My/1, Mz/1
  Constant/1 -> SwitchFx/1, SwitchFz/1, SwitchFy/1
  Fz-AFK/1 -> Fz-Sum/3
  Fz-A/1 -> Fz-Sum/2
  Fz-w/1 -> Fz-Sum/1
  Fx-AFK/1 -> Fx-Sum/3
  Fx-A/1 -> Fx-Sum/2
  Fx-u/1 -> Fx-Sum/1
  w-A-Sum/1 -> Fz-AFK/1, AccelDiff-w/1
  AccelDiff-w/1 -> Fz-A/1
  Vol/1 -> Fx-A/3, Fz-A/2, Fx-AFK/2, Fz-AFK/2, Fy-AFK/2, Fy-A/3
  AccelDiff-x/1 -> Fx-A/1
  V^2-w/1 -> Fz-w/1
  Density/1 -> Fz-w/3, Fx-u/3, Fy-v/3, Fx-A/2, Fz-A/3, Fx-AFK/3, Fz-AFK/3, Fy-AFK/3, Fy-A/2
  half/1 -> Fx-u/2, Fy-v/2, Fz-w/2
  V^2-u/1 -> Fx-u/1
  VelDiff-w/1 -> V-w/1, V^2-w/2
  w-V-Sum/1 -> VelDiff-w/1
  u-V-Sum/1 -> VelDiff-u/1
  Uz/1 -> VelDiff-w/2
  Ux/1 -> VelDiff-u/2
  Uy/1 -> VelDiff-v/2
  Add Vel/1 -> Uz/1, Uy/1, Ux/1
  "dot{U}z"/1 -> AccelDiff-w/2
  x-A-Sum/1 -> AccelDiff-x/1, Fx-AFK/1
  "dot{U}x"/1 -> AccelDiff-x/2
  "dot{U}y"/1 -> AccelDiff-v/2
  ShiftCg/1 -> Zshift/1, MorisonElementIrregular/1(Disp)
  Disp-sl/1 -> ShiftCg/2
  r x 3x3/1 -> ShiftCg/1, "r_{cg} x F"/1
  Rotation3/1(rot[3,1-3]) -> 3x3/3
  Rotation1/1(rot[1,1-3]) -> 3x3/1
  Rotation2/1(rot[2,1-3]) -> 3x3/2
  rot2/1 -> Rotation1/2(rot2), Rotation2/2(rot2), Rotation3/2(rot2)
  rot1/1 -> Rotation1/1(rot1), Rotation2/1(rot1), Rotation3/1(rot1)
  rot3/1 -> Rotation1/3(rot3), Rotation2/3(rot3)
  Disp-sr/1 -> rot1/1, rot2/1, rot3/1
  Disp/1 -> Disp-sr/1, Disp-sl/1
  Vel-sl/1 -> Add Vel/1
  Add Accel/1 -> "dot{U}x"/1, "dot{U}y"/1, "dot{U}z"/1
  Accel-sl/1 -> Add Accel/3
  "dot{w} x r2"/1 -> Add Accel/2
  Accel-sr/1 -> "dot{w} x r2"/1
  Accel/1 -> Accel-sr/1, Accel-sl/1
  r/1 -> w x r/2, "dot{w} x r2"/2, r x 3x3/1
  "Vel-sr "/1 -> w x r/1, w x w x r/1
  w x w x r/1 -> Add Accel/1
  w x r/1 -> w x w x r/2, Add Vel/2
  Vel/1 -> "Vel-sr "/1, Vel-sl/1

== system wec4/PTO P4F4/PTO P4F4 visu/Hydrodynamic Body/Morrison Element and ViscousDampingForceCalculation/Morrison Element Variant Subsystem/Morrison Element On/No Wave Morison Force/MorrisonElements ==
  r : Inport  Partition=on  PartitionDimension=1  PartitionWidth=1
  Vel : Inport  Port=2
  Accel : Inport  Port=3
  Disp : Inport  Port=4
  Area : Inport  Port=5  Partition=on  PartitionDimension=1  PartitionWidth=1
  Cd : Inport  Port=6  Partition=on  PartitionDimension=1  PartitionWidth=1
  Vol : Inport  Port=7  Partition=on  PartitionDimension=1  PartitionWidth=1
  Ca : Inport  Port=8  Partition=on  PartitionDimension=1  PartitionWidth=1
  Time : Inport  Port=9
  3x3 : Concatenate  NumInputs=3  Mode=Multidimensional array
  A x 3x3 : Product  Multiplication=Matrix(*)
  Accel-sl : Selector  InputPortWidth=6  IndexOptions=Index vector (dialog)  Indices=[1 2 3]  OutputSizes=1
  Accel-sr : Selector  InputPortWidth=6  IndexOptions=Index vector (dialog)  Indices=[4 5 6]  OutputSizes=1
  AccelDiff-u : Sum  Inputs=+-
  AccelDiff-v : Sum  Inputs=+-
  AccelDiff-w : Sum  Inputs=+-
  Add Accel : Sum  Inputs=+++
  Add Vel : Sum
  Ax : Selector  InputPortWidth=3  IndexOptions=Index vector (dialog)  Indices=[1]  OutputSizes=1
  Ay : Selector  InputPortWidth=3  IndexOptions=Index vector (dialog)  Indices=[2]  OutputSizes=1
  Az : Selector  InputPortWidth=3  IndexOptions=Index vector (dialog)  Indices=[3]  OutputSizes=1
  Cax : Selector  InputPortWidth=3  IndexOptions=Index vector (dialog)  Indices=[1]  OutputSizes=1
  Cay : Selector  InputPortWidth=3  IndexOptions=Index vector (dialog)  Indices=[2]  OutputSizes=1
  Caz : Selector  InputPortWidth=3  IndexOptions=Index vector (dialog)  Indices=[3]  OutputSizes=1
  Cdx : Selector  InputPortWidth=3  IndexOptions=Index vector (dialog)  Indices=[1]  OutputSizes=1
  Cdy : Selector  InputPortWidth=3  IndexOptions=Index vector (dialog)  Indices=[2]  OutputSizes=1
  Cdz : Selector  InputPortWidth=3  IndexOptions=Index vector (dialog)  Indices=[3]  OutputSizes=1
  Constant : Constant  Value=0
  Density : Constant  Value=simu.rho
  Disp-sl : Selector  InputPortWidth=6  IndexOptions=Index vector (dialog)  Indices=[1 2 3]  OutputSizes=1
  Disp-sr : Selector  InputPortWidth=6  IndexOptions=Index vector (dialog)  Indices=[4 5 6]  OutputSizes=1
  For Each : ForEach  DisableCoverage=on  IndexMode=One-based
  ForceCom : Concatenate  NumInputs=3  ConcatenateDimension=2
  Fout : Concatenate  NumInputs=6  Mode=Multidimensional array  ConcatenateDimension=2
  Fx-A : Product  Inputs=4
  Fx-AFK : Product  Inputs=3
  Fx-Sum : Sum  Inputs=+++
  Fx-V : Product  Inputs=5
  Fx-V1 : Product  Inputs=5
  Fy-A : Product  Inputs=4
  Fy-AFK : Product  Inputs=3
  Fy-Sum : Sum  Inputs=+++
  Fz-A : Product  Inputs=4
  Fz-AFK : Product  Inputs=3
  Fz-Sum : Sum  Inputs=+++
  Fz-w : Product  Inputs=5
  Mx : Selector  InputPortWidth=3  IndexOptions=Index vector (dialog)  Indices=[1]  OutputSizes=1
  My : Selector  InputPortWidth=3  IndexOptions=Index vector (dialog)  Indices=[2]  OutputSizes=1
  Mz : Selector  InputPortWidth=3  IndexOptions=Index vector (dialog)  Indices=[3]  OutputSizes=1
  OrbitalVelocity : Subsystem
  Rotation1 : Subsystem
  Rotation2 : Subsystem
  Rotation3 : Subsystem
  ShiftCg : Sum
  SwitchFx : Switch  Criteria=u2 > Threshold
  SwitchFy : Switch  Criteria=u2 > Threshold
  SwitchFz : Switch  Criteria=u2 > Threshold
  Ux : Selector  InputPortWidth=3  IndexOptions=Index vector (dialog)  Indices=[1]  OutputSizes=1
  Uy : Selector  InputPortWidth=3  IndexOptions=Index vector (dialog)  Indices=[2]  OutputSizes=1
  Uz : Selector  InputPortWidth=3  IndexOptions=Index vector (dialog)  Indices=[3]  OutputSizes=1
  V-u : Abs
  V-v : Abs
  V-w : Abs
  V^2-u : Product
  V^2-v : Product
  V^2-w : Product
  Vel-sl : Selector  InputPortWidth=6  IndexOptions=Index vector (dialog)  Indices=[1 2 3]  OutputSizes=1
  "Vel-sr " : Selector  InputPortWidth=6  IndexOptions=Index vector (dialog)  Indices=[4 5 6]  OutputSizes=1
  VelDiff-u : Sum  Inputs=+-
  VelDiff-v : Sum  Inputs=+-
  VelDiff-w : Sum  Inputs=+-
  Zshift : Selector  InputPortWidth=3  IndexOptions=Index vector (dialog)  Indices=[3]  OutputSizes=1
  abs-Area : Abs
  abs-Ca : Abs
  abs-Cd : Abs
  "dot{U}x" : Selector  InputPortWidth=3  IndexOptions=Index vector (dialog)  Indices=[1]  OutputSizes=1
  "dot{U}y" : Selector  InputPortWidth=3  IndexOptions=Index vector (dialog)  Indices=[2]  OutputSizes=1
  "dot{U}z" : Selector  InputPortWidth=3  IndexOptions=Index vector (dialog)  Indices=[3]  OutputSizes=1
  "dot{w} x r2" : vrlib/Utilities/Cross Product
  half : Constant  Value=1/2
  r x 3x1 : Product  Multiplication=Matrix(*)
  r x 3x2 : Product  Multiplication=Matrix(*)
  r x 3x3 : Product  Multiplication=Matrix(*)
  "r_{cg} x F" : vrlib/Utilities/Cross Product
  rot1 : Selector  InputPortWidth=3  IndexOptions=Index vector (dialog)  Indices=[1]  OutputSizes=1
  rot2 : Selector  InputPortWidth=3  IndexOptions=Index vector (dialog)  Indices=[2]  OutputSizes=1
  rot3 : Selector  InputPortWidth=3  IndexOptions=Index vector (dialog)  Indices=[3]  OutputSizes=1
  w x r : vrlib/Utilities/Cross Product
  w x w x r : vrlib/Utilities/Cross Product
  Force : Outport  PortDimensions=[1 6]  ConcatenationDimension=1
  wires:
  Time/1 -> OrbitalVelocity/2(Time)
  abs-Cd/1 -> r x 3x1/1
  abs-Ca/1 -> Caz/1, Cay/1, Cax/1
  V-w/1 -> V^2-w/1
  Constant/1 -> SwitchFx/1, SwitchFz/1, SwitchFy/1
  Fx-V1/1 -> Fy-Sum/1
  Fy-A/1 -> Fy-Sum/2
  Cay/1 -> Fy-A/4
  AccelDiff-v/1 -> Fy-A/1
  Fy-AFK/1 -> Fy-Sum/3
  Fy-Sum/1 -> SwitchFy/3
  SwitchFy/1 -> ForceCom/2, Fout/2
  Cdy/1 -> Fx-V1/4
  Ay/1 -> Fx-V1/5
  OrbitalVelocity/5(v-V) -> VelDiff-v/1
  VelDiff-v/1 -> V^2-v/2, V-v/1
  V-v/1 -> V^2-v/1
  V^2-v/1 -> Fx-V1/1
  OrbitalVelocity/6(v-A) -> Fy-AFK/1, AccelDiff-v/1
  r x 3x2/1 -> abs-Ca/1
  Ca/1 -> r x 3x2/1
  r x 3x1/1 -> Cdx/1, Cdz/1, Cdy/1
  Cd/1 -> abs-Cd/1
  Cax/1 -> Fx-A/4
  Caz/1 -> Fz-A/4
  Fout/1 -> Force/1
  ForceCom/1 -> "r_{cg} x F"/2
  abs-Area/1 -> Ax/1, Az/1, Ay/1
  A x 3x3/1 -> abs-Area/1
  Cdz/1 -> Fz-w/4
  Cdx/1 -> Fx-V/4
  Ax/1 -> Fx-V/5
  Area/1 -> A x 3x3/1
  Az/1 -> Fz-w/5
  Fz-Sum/1 -> SwitchFz/3
  Fx-Sum/1 -> SwitchFx/3
  SwitchFx/1 -> ForceCom/1, Fout/1
  SwitchFz/1 -> Fout/3, ForceCom/3
  Zshift/1 -> SwitchFz/2, SwitchFx/2, SwitchFy/2
  VelDiff-u/1 -> V^2-u/2, V-u/1
  V-u/1 -> V^2-u/1
  3x3/1 -> r x 3x1/2, r x 3x2/2, r x 3x3/2, A x 3x3/2
  Mz/1 -> Fout/6
  My/1 -> Fout/5
  Mx/1 -> Fout/4
  "r_{cg} x F"/1 -> Mx/1, My/1, Mz/1
  Fz-AFK/1 -> Fz-Sum/3
  Fz-A/1 -> Fz-Sum/2
  Fz-w/1 -> Fz-Sum/1
  Fx-AFK/1 -> Fx-Sum/3
  Fx-A/1 -> Fx-Sum/2
  Fx-V/1 -> Fx-Sum/1
  OrbitalVelocity/4(w-A) -> AccelDiff-w/1, Fz-AFK/1
  AccelDiff-w/1 -> Fz-A/1
  Vol/1 -> Fx-A/3, Fz-A/2, Fx-AFK/2, Fz-AFK/2, Fy-AFK/2, Fy-A/2
  AccelDiff-u/1 -> Fx-A/1
  V^2-w/1 -> Fz-w/1
  Density/1 -> Fx-V/3, Fx-V1/3, Fz-w/3, Fx-A/2, Fz-A/3, Fx-AFK/3, Fz-AFK/3, Fy-AFK/3, Fy-A/3
  half/1 -> Fx-V/2, Fx-V1/2, Fz-w/2
  V^2-u/1 -> Fx-V/1
  VelDiff-w/1 -> V^2-w/2, V-w/1
  OrbitalVelocity/2(w-V) -> VelDiff-w/1
  OrbitalVelocity/1(u-V) -> VelDiff-u/1
  Uz/1 -> VelDiff-w/2
  Ux/1 -> VelDiff-u/2
  Uy/1 -> VelDiff-v/2
  Add Vel/1 -> Ux/1, Uz/1, Uy/1
  "dot{U}z"/1 -> AccelDiff-w/2
  OrbitalVelocity/3(u-A) -> Fx-AFK/1, AccelDiff-u/1
  "dot{U}x"/1 -> AccelDiff-u/2
  "dot{U}y"/1 -> AccelDiff-v/2
  ShiftCg/1 -> OrbitalVelocity/1(Disp), Zshift/1
  Disp-sl/1 -> ShiftCg/2
  r x 3x3/1 -> ShiftCg/1, "r_{cg} x F"/1
  Rotation3/1(rot[3,1-3]) -> 3x3/3
  Rotation1/1(rot[1,1-3]) -> 3x3/1
  Rotation2/1(rot[2,1-3]) -> 3x3/2
  rot2/1 -> Rotation1/2(rot2), Rotation2/2(rot2), Rotation3/2(rot2)
  rot1/1 -> Rotation1/1(rot1), Rotation2/1(rot1), Rotation3/1(rot1)
  rot3/1 -> Rotation1/3(rot3), Rotation2/3(rot3)
  Disp-sr/1 -> rot1/1, rot2/1, rot3/1
  Disp/1 -> Disp-sr/1, Disp-sl/1
  Vel-sl/1 -> Add Vel/1
  Add Accel/1 -> "dot{U}x"/1, "dot{U}y"/1, "dot{U}z"/1
  Accel-sl/1 -> Add Accel/3
  "dot{w} x r2"/1 -> Add Accel/2
  Accel-sr/1 -> "dot{w} x r2"/1
  Accel/1 -> Accel-sr/1, Accel-sl/1
  r/1 -> w x r/2, "dot{w} x r2"/2, r x 3x3/1
  "Vel-sr "/1 -> w x r/1, w x w x r/1
  w x w x r/1 -> Add Accel/1
  w x r/1 -> w x w x r/2, Add Vel/2
  Vel/1 -> "Vel-sr "/1, Vel-sl/1

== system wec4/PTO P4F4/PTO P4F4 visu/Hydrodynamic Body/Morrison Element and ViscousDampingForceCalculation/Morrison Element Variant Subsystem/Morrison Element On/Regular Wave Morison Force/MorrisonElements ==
  r : Inport  Partition=on  PartitionDimension=1  PartitionWidth=1
  Vel : Inport  Port=2
  Accel : Inport  Port=3
  Disp : Inport  Port=4
  Area : Inport  Port=5  Partition=on  PartitionDimension=1  PartitionWidth=1
  Cd : Inport  Port=6  Partition=on  PartitionDimension=1  PartitionWidth=1
  Vol : Inport  Port=7  Partition=on  PartitionDimension=1  PartitionWidth=1
  Ca : Inport  Port=8  Partition=on  PartitionDimension=1  PartitionWidth=1
  Time : Inport  Port=9
  3x3 : Concatenate  NumInputs=3  Mode=Multidimensional array
  A x 3x3 : Product  Multiplication=Matrix(*)
  Accel-sl : Selector  InputPortWidth=6  IndexOptions=Index vector (dialog)  Indices=[1 2 3]  OutputSizes=1
  Accel-sr : Selector  InputPortWidth=6  IndexOptions=Index vector (dialog)  Indices=[4 5 6]  OutputSizes=1
  AccelDiff-u : Sum  Inputs=+-
  AccelDiff-v : Sum  Inputs=+-
  AccelDiff-w : Sum  Inputs=+-
  Add Accel : Sum  Inputs=+++
  Add Vel : Sum
  Ax : Selector  InputPortWidth=3  IndexOptions=Index vector (dialog)  Indices=[1]  OutputSizes=1
  Ay : Selector  InputPortWidth=3  IndexOptions=Index vector (dialog)  Indices=[2]  OutputSizes=1
  Az : Selector  InputPortWidth=3  IndexOptions=Index vector (dialog)  Indices=[3]  OutputSizes=1
  Cax : Selector  InputPortWidth=3  IndexOptions=Index vector (dialog)  Indices=[1]  OutputSizes=1
  Cay : Selector  InputPortWidth=3  IndexOptions=Index vector (dialog)  Indices=[2]  OutputSizes=1
  Caz : Selector  InputPortWidth=3  IndexOptions=Index vector (dialog)  Indices=[3]  OutputSizes=1
  Cdx : Selector  InputPortWidth=3  IndexOptions=Index vector (dialog)  Indices=[1]  OutputSizes=1
  Cdy : Selector  InputPortWidth=3  IndexOptions=Index vector (dialog)  Indices=[2]  OutputSizes=1
  Cdz : Selector  InputPortWidth=3  IndexOptions=Index vector (dialog)  Indices=[3]  OutputSizes=1
  Constant : Constant  Value=0
  Density : Constant  Value=simu.rho
  Disp-sl : Selector  InputPortWidth=6  IndexOptions=Index vector (dialog)  Indices=[1 2 3]  OutputSizes=1
  Disp-sr : Selector  InputPortWidth=6  IndexOptions=Index vector (dialog)  Indices=[4 5 6]  OutputSizes=1
  For Each : ForEach  DisableCoverage=on  IndexMode=One-based
  ForceCom : Concatenate  NumInputs=3  ConcatenateDimension=2
  Fout : Concatenate  NumInputs=6  Mode=Multidimensional array  ConcatenateDimension=2
  Fx-A : Product  Inputs=4
  Fx-AFK : Product  Inputs=3
  Fx-Sum : Sum  Inputs=+++
  Fx-V : Product  Inputs=5
  Fx-V1 : Product  Inputs=5
  Fy-A : Product  Inputs=4
  Fy-AFK : Product  Inputs=3
  Fy-Sum : Sum  Inputs=+++
  Fz-A : Product  Inputs=4
  Fz-AFK : Product  Inputs=3
  Fz-Sum : Sum  Inputs=+++
  Fz-w : Product  Inputs=5
  Mx : Selector  InputPortWidth=3  IndexOptions=Index vector (dialog)  Indices=[1]  OutputSizes=1
  My : Selector  InputPortWidth=3  IndexOptions=Index vector (dialog)  Indices=[2]  OutputSizes=1
  Mz : Selector  InputPortWidth=3  IndexOptions=Index vector (dialog)  Indices=[3]  OutputSizes=1
  OrbitalVelocity : Subsystem
  Rotation1 : Subsystem
  Rotation2 : Subsystem
  Rotation3 : Subsystem
  ShiftCg : Sum
  SwitchFx : Switch  Criteria=u2 > Threshold
  SwitchFy : Switch  Criteria=u2 > Threshold
  SwitchFz : Switch  Criteria=u2 > Threshold
  Ux : Selector  InputPortWidth=3  IndexOptions=Index vector (dialog)  Indices=[1]  OutputSizes=1
  Uy : Selector  InputPortWidth=3  IndexOptions=Index vector (dialog)  Indices=[2]  OutputSizes=1
  Uz : Selector  InputPortWidth=3  IndexOptions=Index vector (dialog)  Indices=[3]  OutputSizes=1
  V-u : Abs
  V-v : Abs
  V-w : Abs
  V^2-u : Product
  V^2-v : Product
  V^2-w : Product
  Vel-sl : Selector  InputPortWidth=6  IndexOptions=Index vector (dialog)  Indices=[1 2 3]  OutputSizes=1
  "Vel-sr " : Selector  InputPortWidth=6  IndexOptions=Index vector (dialog)  Indices=[4 5 6]  OutputSizes=1
  VelDiff-u : Sum  Inputs=+-
  VelDiff-v : Sum  Inputs=+-
  VelDiff-w : Sum  Inputs=+-
  Zshift : Selector  InputPortWidth=3  IndexOptions=Index vector (dialog)  Indices=[3]  OutputSizes=1
  abs-Area : Abs
  abs-Ca : Abs
  abs-Cd : Abs
  "dot{U}x" : Selector  InputPortWidth=3  IndexOptions=Index vector (dialog)  Indices=[1]  OutputSizes=1
  "dot{U}y" : Selector  InputPortWidth=3  IndexOptions=Index vector (dialog)  Indices=[2]  OutputSizes=1
  "dot{U}z" : Selector  InputPortWidth=3  IndexOptions=Index vector (dialog)  Indices=[3]  OutputSizes=1
  "dot{w} x r2" : vrlib/Utilities/Cross Product
  half : Constant  Value=1/2
  r x 3x1 : Product  Multiplication=Matrix(*)
  r x 3x2 : Product  Multiplication=Matrix(*)
  r x 3x3 : Product  Multiplication=Matrix(*)
  "r_{cg} x F" : vrlib/Utilities/Cross Product
  rot1 : Selector  InputPortWidth=3  IndexOptions=Index vector (dialog)  Indices=[1]  OutputSizes=1
  rot2 : Selector  InputPortWidth=3  IndexOptions=Index vector (dialog)  Indices=[2]  OutputSizes=1
  rot3 : Selector  InputPortWidth=3  IndexOptions=Index vector (dialog)  Indices=[3]  OutputSizes=1
  w x r : vrlib/Utilities/Cross Product
  w x w x r : vrlib/Utilities/Cross Product
  Force : Outport  PortDimensions=[1 6]  ConcatenationDimension=1
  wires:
  Time/1 -> OrbitalVelocity/2(Time)
  abs-Cd/1 -> r x 3x1/1
  abs-Ca/1 -> Caz/1, Cay/1, Cax/1
  V-w/1 -> V^2-w/1
  Constant/1 -> SwitchFx/1, SwitchFz/1, SwitchFy/1
  Fx-V1/1 -> Fy-Sum/1
  Fy-A/1 -> Fy-Sum/2
  Cay/1 -> Fy-A/4
  AccelDiff-v/1 -> Fy-A/1
  Fy-AFK/1 -> Fy-Sum/3
  Fy-Sum/1 -> SwitchFy/3
  SwitchFy/1 -> ForceCom/2, Fout/2
  Cdy/1 -> Fx-V1/4
  Ay/1 -> Fx-V1/5
  OrbitalVelocity/5(v-V) -> VelDiff-v/1
  VelDiff-v/1 -> V^2-v/2, V-v/1
  V-v/1 -> V^2-v/1
  V^2-v/1 -> Fx-V1/1
  OrbitalVelocity/6(v-A) -> Fy-AFK/1, AccelDiff-v/1
  r x 3x2/1 -> abs-Ca/1
  Ca/1 -> r x 3x2/1
  r x 3x1/1 -> Cdx/1, Cdz/1, Cdy/1
  Cd/1 -> abs-Cd/1
  Cax/1 -> Fx-A/4
  Caz/1 -> Fz-A/4
  Fout/1 -> Force/1
  ForceCom/1 -> "r_{cg} x F"/2
  abs-Area/1 -> Ax/1, Az/1, Ay/1
  A x 3x3/1 -> abs-Area/1
  Cdz/1 -> Fz-w/4
  Cdx/1 -> Fx-V/4
  Ax/1 -> Fx-V/5
  Area/1 -> A x 3x3/1
  Az/1 -> Fz-w/5
  Fz-Sum/1 -> SwitchFz/3
  Fx-Sum/1 -> SwitchFx/3
  SwitchFx/1 -> ForceCom/1, Fout/1
  SwitchFz/1 -> Fout/3, ForceCom/3
  Zshift/1 -> SwitchFz/2, SwitchFx/2, SwitchFy/2
  VelDiff-u/1 -> V^2-u/2, V-u/1
  V-u/1 -> V^2-u/1
  3x3/1 -> r x 3x1/2, r x 3x2/2, r x 3x3/2, A x 3x3/2
  Mz/1 -> Fout/6
  My/1 -> Fout/5
  Mx/1 -> Fout/4
  "r_{cg} x F"/1 -> Mx/1, My/1, Mz/1
  Fz-AFK/1 -> Fz-Sum/3
  Fz-A/1 -> Fz-Sum/2
  Fz-w/1 -> Fz-Sum/1
  Fx-AFK/1 -> Fx-Sum/3
  Fx-A/1 -> Fx-Sum/2
  Fx-V/1 -> Fx-Sum/1
  OrbitalVelocity/4(w-A) -> AccelDiff-w/1, Fz-AFK/1
  AccelDiff-w/1 -> Fz-A/1
  Vol/1 -> Fx-A/3, Fz-A/2, Fx-AFK/2, Fz-AFK/2, Fy-AFK/2, Fy-A/2
  AccelDiff-u/1 -> Fx-A/1
  V^2-w/1 -> Fz-w/1
  Density/1 -> Fx-V/3, Fx-V1/3, Fz-w/3, Fx-A/2, Fz-A/3, Fx-AFK/3, Fz-AFK/3, Fy-AFK/3, Fy-A/3
  half/1 -> Fx-V/2, Fx-V1/2, Fz-w/2
  V^2-u/1 -> Fx-V/1
  VelDiff-w/1 -> V^2-w/2, V-w/1
  OrbitalVelocity/2(w-V) -> VelDiff-w/1
  OrbitalVelocity/1(u-V) -> VelDiff-u/1
  Uz/1 -> VelDiff-w/2
  Ux/1 -> VelDiff-u/2
  Uy/1 -> VelDiff-v/2
  Add Vel/1 -> Ux/1, Uz/1, Uy/1
  "dot{U}z"/1 -> AccelDiff-w/2
  OrbitalVelocity/3(u-A) -> Fx-AFK/1, AccelDiff-u/1
  "dot{U}x"/1 -> AccelDiff-u/2
  "dot{U}y"/1 -> AccelDiff-v/2
  ShiftCg/1 -> OrbitalVelocity/1(Disp), Zshift/1
  Disp-sl/1 -> ShiftCg/2
  r x 3x3/1 -> ShiftCg/1, "r_{cg} x F"/1
  Rotation3/1(rot[3,1-3]) -> 3x3/3
  Rotation1/1(rot[1,1-3]) -> 3x3/1
  Rotation2/1(rot[2,1-3]) -> 3x3/2
  rot2/1 -> Rotation1/2(rot2), Rotation2/2(rot2), Rotation3/2(rot2)
  rot1/1 -> Rotation1/1(rot1), Rotation2/1(rot1), Rotation3/1(rot1)
  rot3/1 -> Rotation1/3(rot3), Rotation2/3(rot3)
  Disp-sr/1 -> rot1/1, rot2/1, rot3/1
  Disp/1 -> Disp-sr/1, Disp-sl/1
  Vel-sl/1 -> Add Vel/1
  Add Accel/1 -> "dot{U}x"/1, "dot{U}y"/1, "dot{U}z"/1
  Accel-sl/1 -> Add Accel/3
  "dot{w} x r2"/1 -> Add Accel/2
  Accel-sr/1 -> "dot{w} x r2"/1
  Accel/1 -> Accel-sr/1, Accel-sl/1
  r/1 -> w x r/2, "dot{w} x r2"/2, r x 3x3/1
  "Vel-sr "/1 -> w x r/1, w x w x r/1
  w x w x r/1 -> Add Accel/1
  w x r/1 -> w x w x r/2, Add Vel/2
  Vel/1 -> "Vel-sr "/1, Vel-sl/1
